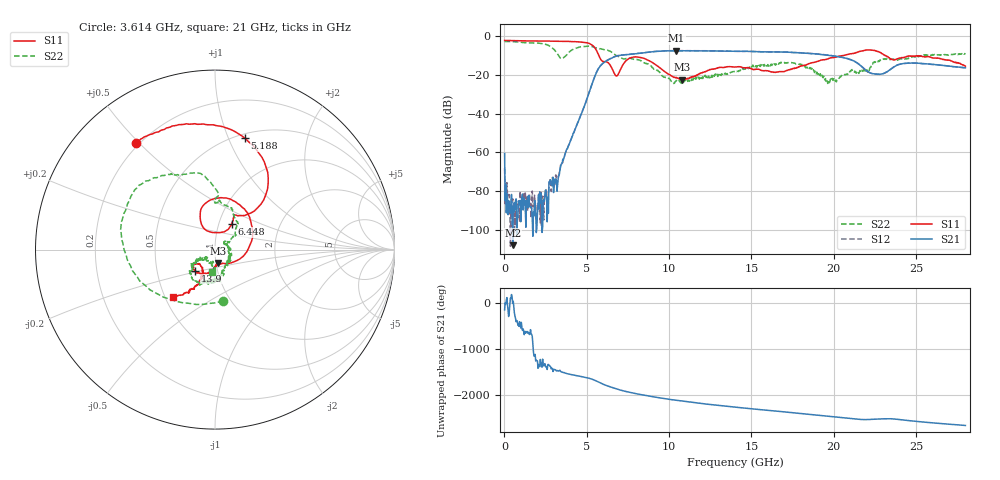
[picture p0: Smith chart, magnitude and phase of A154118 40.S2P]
!  2-Port S-parameters saved by WinCal
! VAR MeasName=S-Parameters (CALIBRATED_DATA) read from VNA (N5230A)
! VAR MeasDate=2015-9-10 14:37:30
! VAR NAME=A154118 40
! VAR FILENAME=A154118 40.S2P
! VAR DATE=2015-9-10 14:37:30
! VAR PHYS_PORTS=1,2
# Hz S DB R 50
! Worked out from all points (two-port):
!   801 points, 10 MHz to 28 GHz, reference 50 ohm
!   highest |S21| = -7.45 dB at 10.44 GHz (marker M1); lowest = -108.0 dB at 499.8 MHz (marker M2)
!   |S21| within 3 dB of the highest: 6.72 GHz to 20.2 GHz (13.48 GHz wide, 100 % of centre)
!   lowest |S11| = -22.3 dB at 10.79 GHz (marker M3), VSWR 1.17, Z = 51.2 - j7.66 ohm
!   |S11| at or under -10 dB: 5.736 GHz to 20.54 GHz (14.8 GHz wide, 113 % of centre); 23.13 GHz to end of sweep
!   |S22| runs from -24.4 to -2.7 dB; largest |S21 - S12| = 0.0086
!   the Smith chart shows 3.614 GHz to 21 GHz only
!   S11 on the Smith chart (normalised r, x): 3.614 GHz: 0.19, +0.49; 5.188 GHz: 0.54, +1.15; 6.448 GHz: 1.15, +0.34; 13.9 GHz: 0.78, -0.19; 21 GHz: 0.55, -0.33
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1e7  -2.15 179.7  -60.53 -140.2  -68.16 15.1  -2.67 179.8
1.849375e8  -2.16 177.2  -83.67 -31.2  -81.87 169.6  -2.69 175.5
4.99825e8  -2.24 172.8  -108.00 1.7  -83.99 109.6  -2.77 167.8
2.599075e9  -2.44 144.8  -95.86 -8.3  -86.02 49.7  -4.40 95.7
3.158875e9  -2.51 135.5  -74.86 -40.2  -74.28 -31.4  -8.27 31.9
3.613712e9  -2.62 126.5  -62.78 -73.9  -63.02 -81.3  -10.83 -81.0
4.698325e9  -3.04 97.9  -39.54 -165.1  -39.53 -165.0  -5.33 165.1
5.18815e9  -3.84 74.9  -27.87 155.3  -27.84 155.4  -5.15 140.7
6.4477e9  -15.33 57.1  -11.48 -32.0  -11.42 -32.0  -7.85 97.3
6.832562e9  -20.46 93.1  -10.12 -77.0  -10.08 -77.2  -10.14 86.3
7.917175e9  -10.68 79.6  -9.07 -172.9  -9.04 -173.2  -11.88 75.6
9.351662e9  -15.64 -11.2  -7.77 94.4  -7.70 94.2  -18.05 35.9
1.043628e10  -21.22 -68.7  -7.45 35.1  -7.42 34.7  -23.07 28.0
1.078615e10  -22.34 -77.1  -7.49 18.4  -7.40 17.7  -23.72 31.4
1.390004e10  -15.87 -133.1  -7.74 -109.9  -7.75 -110.6  -18.27 -64.4
1.4005e10  -15.85 -135.5  -7.77 -113.8  -7.75 -114.4  -18.24 -67.1
1.627919e10  -18.40 -138.3  -8.08 167.2  -8.07 166.5  -14.37 -105.6
1.869332e10  -13.63 -115.2  -8.93 83.7  -8.93 83.2  -16.90 -142.8
1.967298e10  -11.59 -122.5  -9.86 49.3  -9.69 48.5  -23.47 -142.4
2.10025e10  -9.11 -131.4  -12.02 -0.3  -11.95 -1.2  -18.03 -96.9
2.334666e10  -11.06 -177.0  -17.69 -7.3  -17.67 -8.3  -12.13 -93.4
2.8e10  -15.45 167.6  -16.24 -155.6  -16.31 -156.8  -8.74 -119.8
